(* Logix 5000 AddOnInstructionDefinition export ACS_FORCE_MOVE; software revision 20.01 *)

ADD_ON_INSTRUCTION ACS_FORCE_MOVE   (* revision 2.0, vendor Tolomatic, Inc *)
// Move to an Absolute Position using Force Move logic
VAR_INPUT
   Position : REAL; {required}   // Absolute Position
   Acceleration : REAL; {required}   // Trajectory Acceleration
   Deceleration : REAL; {required}   // Trajectory Deceleration
   Velocity : REAL; {required}   // Trajectory Constant Velocity
   Force : REAL; {required}   // Force Limit (Percent)
END_VAR
VAR_IN_OUT
   DriveMoveSelect : SINT; {required}   // ACS.O.MOVESELECT
   DriveTargetPos : REAL; {required}   // ACS.O.TARGET_0_POS
   DriveTargetVel : REAL; {required}   // ACS.O.TARGET_0_VEL
   DriveTargetAcc : REAL; {required}   // ACS.O.TARGET_0_ACC
   DriveTargetDec : REAL; {required}   // ACS.O.TARGET_0_DEC
   DriveTargetForce : REAL; {required}   // ACS.O.TARGET_0_FORCE
   DriveTargetMotionType : DINT; {required}   // ACS.O.TARGET_0_MOTION_TYPE
END_VAR

ROUTINE Logic   (* ladder *)
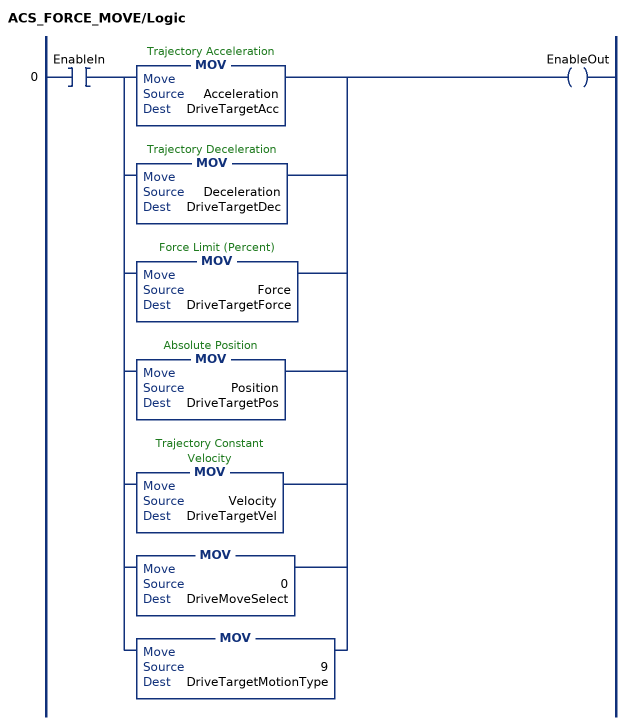
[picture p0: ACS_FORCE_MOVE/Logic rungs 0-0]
   0: XIC(EnableIn)[MOV(Acceleration,DriveTargetAcc) ,MOV(Deceleration,DriveTargetDec) ,MOV(Force,DriveTargetForce) ,MOV(Position,DriveTargetPos) ,MOV(Velocity,DriveTargetVel) ,MOV(0,DriveMoveSelect) ,MOV(9,DriveTargetMotionType) ]OTE(EnableOut);
END_ROUTINE
END_ADD_ON_INSTRUCTION
